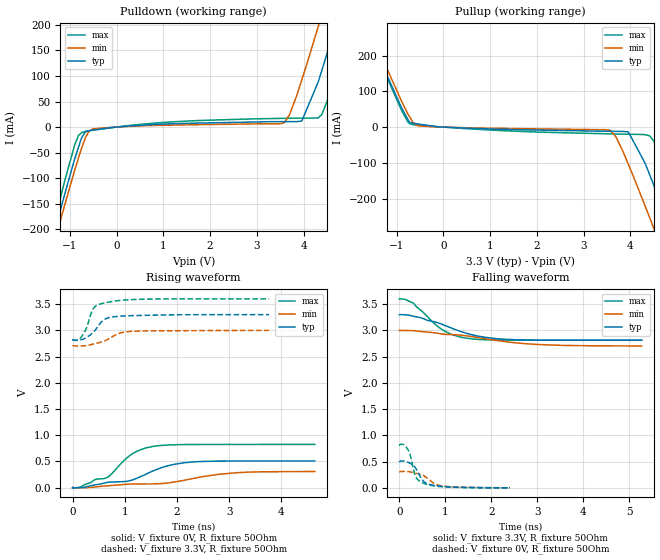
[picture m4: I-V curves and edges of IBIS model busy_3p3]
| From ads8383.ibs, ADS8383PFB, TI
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|   busy_3p3 Model
[Model]   busy_3p3
Model_type   Output
Polarity   Non-Inverting
Vmeas = 1.65
Vref = 1.65
Cref = 10pF
Rref = 50
|   typ   min   max
|   (nom PVT)   (fast PVT)   (slow PVT)
|C_comp from frequency sweep method (F=500KHz)
|C_comp   2.199e-12   2.061e-12   2.322e-12
|ON state : BUFFER OUTPUT TURNED HIGH
|C_comp   2.199e-12   2.061e-12   2.322e-12
|OFF state: BUFFER OUTPUT TURNED LOW
|C_comp   2.277e-12   2.150e-12   2.385e-12
|C_comp from LC tank measurement(L=1nH)
|Resonant Frequency(Hz)   6.440e+09   6.690e+09   6.160e+09
 C_comp   6.114e-13   5.665e-13   6.682e-13
|ON state : BUFFER OUTPUT TURNED HIGH
|Resonant Frequency(Hz)   6.440e+09   6.690e+09   6.160e+09
|C_comp   6.114e-13   5.665e-13   6.682e-13
|OFF state: BUFFER OUTPUT TURNED LOW
|Resonant Frequency(Hz)   6.460e+09   6.740e+09   6.170e+09
|C_comp   6.076e-13   5.582e-13   6.660e-13
| Where nom  PVT is Nominal Process, 3.3V, 35C
|   Fast PVT is Strong Process,  3.6V, -40C
|   Slow PVT is Weak Process,   3V, 95C
[Voltage Range]   3.3   3   3.6
|Ambient Temperature   25   85   -40
|Junction Temperature
[Temperature Range]   35   95   -40
[Pullup Reference]   3.3   3   3.6
[Pulldown Reference]   0   0   0
[Power Clamp Reference]   3.3   3   3.6
[GND Clamp Reference]   0   0   0
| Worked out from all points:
|   slope of the pulldown table from 0 to 0.495 V, typ, clamps not added: 146 ohm
|   slope of the pullup table from 0 to 0.495 V, typ, clamps not added: 169 ohm
|   falling waveform, V_fixture 3.3V, R_fixture 50Ohm: 20-80 % time 1.03ns typ, 1.67ns min, 638ps max; typ from 3.3 V to 2.81 V
|   rising waveform, V_fixture 0V, R_fixture 50Ohm: 20-80 % time 1.12ns typ, 1.76ns min, 691ps max; typ from 0 V to 0.508 V
|   rising waveform, V_fixture 3.3V, R_fixture 50Ohm: 20-80 % time 267ps typ, 392ps min, 190ps max; typ from 2.81 V to 3.3 V
|   falling waveform, V_fixture 0V, R_fixture 50Ohm: 20-80 % time 231ps typ, 321ps min, 168ps max; typ from 0.509 V to 0.002 V
[Pulldown]
|   Voltage   I(typ)   I(min)   I(max)
-3.3V     -901.9mA   -899.7mA   -920.7mA
-1.512V   -269.9mA   -286.5mA   -251.3mA
-1.179V   -155.1mA   -175.4mA   -130.7mA
-813.6mV  -39.4mA    -60.27mA   -16.23mA
-660mV    -8.008mA   -19.76mA   -8.841mA
-504mV    -5.972mA   -3.518mA   -6.081mA
3.591V    10.6mA     8.904mA    17.1mA
3.963V    11.8mA     92.29mA    17.53mA
4.313V    87.92mA    195.9mA    17.95mA
4.723V    212.2mA    323.5mA    114.3mA
5.101V    329.4mA    442.2mA    231.1mA
6.6V      803.1mA    913.1mA    706.9mA
[Pullup]
|   Voltage   I(typ)   I(min)   I(max)
-3.3V     803mA      818.9mA    802.7mA
-1.588V   262mA      280.3mA    257.9mA
-759.6mV  20.97mA    36.51mA    14.2mA
-519mV    8.274mA    3.057mA    5.171mA
3.576V    -11.8mA    -10.03mA   -19.03mA
3.957V    -13.57mA   -104.1mA   -20.08mA
4.417V    -134.8mA   -254.9mA   -24.77mA
4.496V    -161.3mA   -281.4mA   -38.6mA
4.68V     -225mA     -343.5mA   -96.22mA
5.026V    -345.1mA   -462.2mA   -219.9mA
5.263V    -427.8mA   -543.9mA   -308.8mA
6.6V      -901.9mA   -1.003A    -807.7mA
[Ramp]
R_load = 50
|   typ   min   max
dV/dt_r   0.305323/1.11588e-09   0.186027/1.75466e-09   0.4952/6.9199e-10
dV/dt_f   0.291841/1.03212e-09   0.17745/1.67359e-09   0.471351/6.37271e-10
[Falling Waveform]
V_fixture = 3.3V
V_fixture_min = 3V
V_fixture_max = 3.6V
R_fixture = 50Ohm
|   Time   V(typ)   V(min)   V(max)
0s        3.3V       3V         3.6V
132ps     3.298V     3V         3.589V
296ps     3.273V     2.996V     3.523V
760ps     3.165V     2.955V     3.131V
968ps     3.104V     2.928V     2.996V
1.442ns   2.95V      2.9V       2.855V
1.828ns   2.875V     2.848V     2.824V
2.508ns   2.824V     2.766V     2.814V
3.554ns   2.814V     2.716V     2.814V
5.264ns   2.814V     2.705V     2.814V
[Rising Waveform]
V_fixture = 0V
V_fixture_min = 0V
V_fixture_max = 0V
R_fixture = 50Ohm
|   Time   V(typ)   V(min)   V(max)
0s        2.667nV    4.843nV    2.533nV
136ps     1.364mV    42.26uV    7.396mV
434ps     54.14mV    12.9mV     154.8mV
666ps     101mV      36.7mV     196.5mV
1.136ns   144.8mV    69.28mV    639.8mV
1.54ns    319mV      73.19mV    786.5mV
1.856ns   425.5mV    94.26mV    815.9mV
2.296ns   490.2mV    173.5mV    823.9mV
3.144ns   508.6mV    285.6mV    825mV
4.642ns   508.3mV    309.3mV    825.3mV
[Rising Waveform]
V_fixture = 3.3V
V_fixture_min = 3V
V_fixture_max = 3.6V
R_fixture = 50Ohm
|   Time   V(typ)   V(min)   V(max)
0s        2.814V     2.704V     2.814V
106ps     2.811V     2.702V     2.819V
188ps     2.826V     2.703V     2.901V
264ps     2.864V     2.711V     3.038V
364ps     2.933V     2.731V     3.346V
424ps     2.992V     2.745V     3.447V
608ps     3.206V     2.798V     3.522V
876ps     3.267V     2.936V     3.567V
1.114ns   3.278V     2.98V      3.585V
3.766ns   3.3V       3V         3.6V
[Falling Waveform]
V_fixture = 0V
V_fixture_min = 0V
V_fixture_max = 0V
R_fixture = 50Ohm
|   Time   V(typ)   V(min)   V(max)
0s        508.9mV    310.1mV    825.4mV
100ps     512.7mV    313.7mV    819.7mV
182ps     491.2mV    310.7mV    733.8mV
230ps     467.9mV    305mV      638.7mV
326ps     404.9mV    285.5mV    282.3mV
356ps     371.8mV    279mV      212.1mV
536ps     116mV      229.3mV    84.9mV
770ps     46.99mV    79.04mV    36.35mV
990ps     24.9mV     29.19mV    18.48mV
2.402ns   1.592mV    2.581mV    773.9uV
